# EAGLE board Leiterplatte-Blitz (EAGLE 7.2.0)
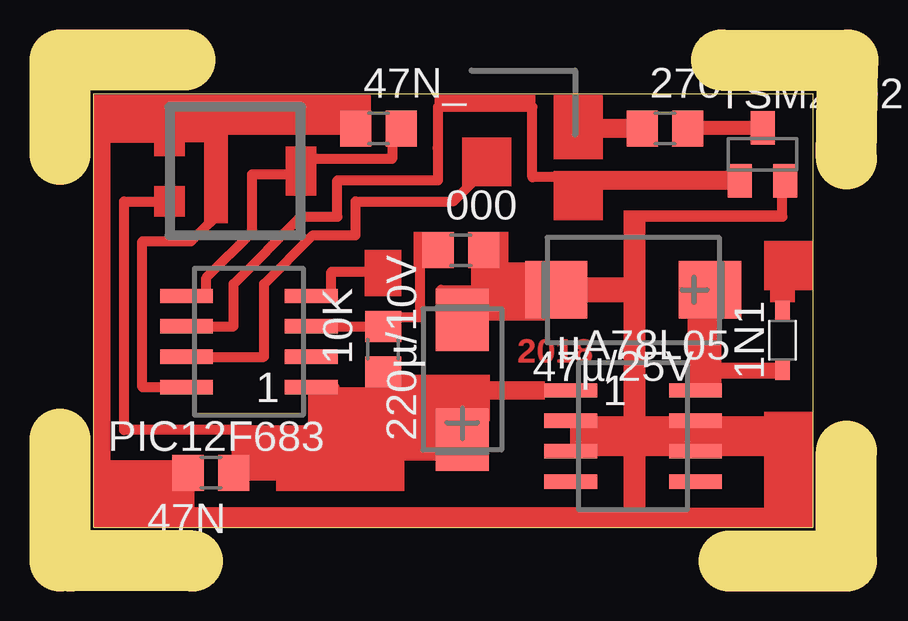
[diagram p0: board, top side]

Size 32.83 x 20.89 mm. Coordinates in mm from the lower left corner, seen from the top.
Outline: 5.53,0 0.44,0
Outline: 0,0 0,5.08
Outline: 27.88,0 32.77,0 32.77,4.57
Outline: 5.21,20.89 0,20.89 0,16.95
Outline: 32.77,16.76 32.83,20.83
Outline: 27.56,20.89 32.83,20.89
Outline: 1.4,1.4 31.37,1.4 31.37,19.49 1.4,19.49 1.4,1.4
Copper layers (1*16): Top 0.035mm / dielectric 1.5mm / Bottom 0.035mm
Design rules "default": minimum track width 10mil, minimum drill 24mil, track to track 8mil, track to pad 8mil, pad to pad 8mil, via to via 8mil, smd to smd 8mil, copper to edge 40mil, drill to drill 8mil, minimum pad ring 10mil, minimum via ring 8mil, stop-mask expansion 4mil, vias tented up to drill 0mil, thermal gap 10mil

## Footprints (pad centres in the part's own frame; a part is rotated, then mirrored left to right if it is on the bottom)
R0805 = smd 1.3 x 1.5: 1 -0.95,0; 2 0.95,0
SOD323R_INFINEON = smd 0.8 x 0.6: A 1.25,0; C -1.25,0
CT7343 = smd 2.6 x 2.4: + -3.2,0; - 3.2,0
CT6032 = smd 2.6 x 2.2: + -2.5,0; - 2.5,0
SOP08 = smd 0.6 x 2.2: 1 -1.905,-2.6; 2 -0.635,-2.6; 3 0.635,-2.6; 4 1.905,-2.6; 5 1.905,2.6; 6 0.635,2.6; 7 -0.635,2.6; 8 -1.905,2.6
SOT23 = smd 1 x 1.4: 1 -0.95,-1.1; 2 0.95,-1.1; 3 0,1.1

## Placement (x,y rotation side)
000  [R0805]  16.7,12.95 0 top
1N1  [SOD323R_INFINEON]  30.1,9.21 90 top
10K  [R0805]  13.46,8.83 90 top
47N  [R0805]  6.29,3.68 180 top
47N_  [R0805]  13.27,18.03 0 top
47µ/25V  [CT7343]  23.88,11.3 180 top
220µ/10V  [CT6032]  16.76,7.56 90 top
270  [R0805]  25.21,18.03 0 top
PIC12F683  [SOP08]  7.87,9.14 90 top
TSM2302  [SOT23]  29.27,16.95 0 top
µA78L05  [SOP08]  23.88,5.21 270 top

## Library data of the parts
000 10K 47N 47N_ 47µ/25V 220µ/10V 270 PIC12F683 TSM2302 µA78L05 = smd-ipc
1N1 = diode

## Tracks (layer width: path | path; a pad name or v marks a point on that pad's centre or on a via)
S$1
  Top 0.406: 11.43,6.6 12.83,6.6 | 11.43,6.6 11.43,7.24 | 10.54,7.24 10.54,6.6 | 10.54,6.6 10.54,3.56 | 10.54,3.56 7.37,3.56 | 7.37,3.56 7.24,3.68 | 7.37,3.56 7.37,5.46 | 7.37,5.46 2.67,5.46 2.67,14.99 4.57,14.99 | 11.43,6.6 10.54,6.6 | 7.37,5.46 10.67,5.46 | 10.54,3.56 13.97,3.56 13.97,5.08
S$2
  Top 0.406: 11.3,9.78 13.21,9.78
S$3
  Top 0.406: 30.1,10.54 30.1,12.32
S$4
  Top 0.406: 28.19,15.88 21.72,15.88
S$5
  Top 0.406: 27.05,5.84 29.97,5.84 29.97,4.57 23.88,4.57 | 23.88,4.57 21.46,4.57 21.46,5.84 26.16,5.84 | 23.88,4.57 23.88,2.03 | 23.88,2.03 4.95,2.03 | 4.95,2.03 4.95,3.94 | 4.95,2.03 1.91,2.03 1.91,17.65 4.57,17.65 | 23.88,2.03 29.72,2.03
S$6
  Top 0.406: 27.05,10.54 27.05,7.87 | 27.05,7.87 27.05,7.11 | 30.1,7.87 27.05,7.87
S$7
  Top 0.406: 20.7,7.11 16.76,7.11 16.76,5.97 | 16.76,5.97 16.76,4.32 | 16.76,5.97 12.83,5.97
S$8
  Top 0.406: 30.1,15.75 30.1,14.35 23.88,14.35 23.88,11.3 15.88,11.3 16.76,9.27
S$9
  Top 0.406: 6.1,11.05 6.1,11.81 8,13.72 8,16.13 10.03,16.13
S$11
  Top 0.406: 4.32,7.24 3.43,7.24 3.43,13.34 5.46,13.34 5.97,13.84 6.22,14.1 | 6.22,14.1 6.22,17.65 | 6.22,17.65 4.83,17.65 | 6.22,17.65 6.22,18.54 11.94,18.54 | 6.22,14.1 6.48,14.35
S$12
  Top 0.406: 17.65,13.08 17.65,11.05
S$13
  Top 0.406: 15.62,13.34 16,13.34
S$14
  Top 0.406: 14.99,13.34 14.99,10.16 13.72,10.16
S$15
  Top 0.406: 20.95,15.37 21.08,15.49
S$16
  Top 0.406: 13.84,17.65 13.84,16.76 10.16,16.76
S$17
  Top 0.406: 6.22,9.78 7.24,9.78 7.24,11.56 10.03,14.35 11.56,14.35 11.56,15.88 15.75,15.88 15.75,17.14 15.75,17.27 15.75,18.92 19.68,18.92 19.68,16 20.95,16
S$18
  Top 0.406: 26.16,18.16 29.08,18.16
S$19
  Top 0.406: 24.26,18.03 21.72,18.03
S$20
  Top 0.406: 6.1,8.51 8.51,8.51 8.51,11.56 10.54,13.59 12.32,13.59 12.32,14.99 16.26,14.99
S$21
  Top 0.406: 16.38,14.99 18.03,16.64
S$22
  Top 0.406: 11.3,11.05 11.3,12.06 13.08,12.06
(copper drawn outside any net)
  shapes: Top area x49

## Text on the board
Top: 2018
tDocu: LED-Anode | 5K | Data | Clock | Vpp | +9V bis +22V | Masse | +5V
